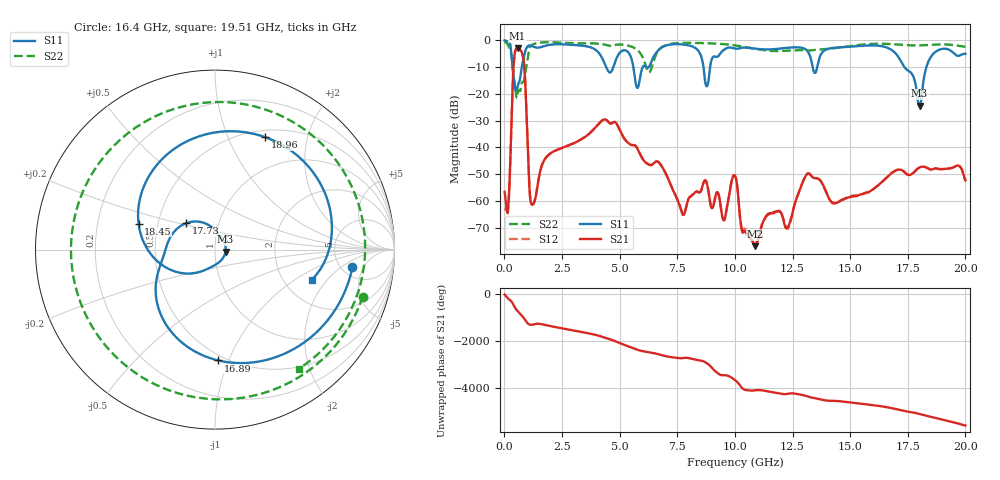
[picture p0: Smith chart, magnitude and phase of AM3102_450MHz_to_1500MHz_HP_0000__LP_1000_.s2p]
!Agilent Technologies,E8364B,MY43040894,A.07.50.67
!Agilent E8364B: A.07.50.67
!Date: Thursday, January 11, 2018 05:16:45
!Correction: S11(Full 2 Port(1,2))
!S21(Full 2 Port(1,2))
!S12(Full 2 Port(1,2))
!S22(Full 2 Port(1,2))
!S2P File: Measurements: S11, S21, S12, S22:
# Hz S  dB  R 50
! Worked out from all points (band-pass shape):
!   1601 points, 10 MHz to 20 GHz, reference 50 ohm
!   highest |S21| = -3.03 dB at 572.2 MHz (marker M1); lowest = -76.8 dB at 10.89 GHz (marker M2)
!   |S21| within 3 dB of the highest: 433.8 MHz to 803.5 MHz (369.7 MHz wide, 59.8 % of centre)
!   lowest |S11| = -24.4 dB at 18.01 GHz (marker M3), VSWR 1.13, Z = 56.2 - j1.22 ohm
!   |S11| at or under -10 dB: 355.7 MHz to 753.7 MHz (398.1 MHz wide, 71.8 % of centre); 5.595 GHz to 6.003 GHz (408.2 MHz wide, 7.04 % of centre); 17.35 GHz to 18.31 GHz (953.5 MHz wide, 5.35 % of centre)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
!   |S22| runs from -21.4 to -0.5 dB; largest |S21 - S12| = 0.0016
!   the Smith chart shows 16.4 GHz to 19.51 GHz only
!   S11 on the Smith chart (normalised r, x): 16.4 GHz: 6.26, -3.06; 16.89 GHz: 0.46, -0.92; 17.73 GHz: 0.70, +0.21; 18.45 GHz: 0.39, +0.14; 18.96 GHz: 0.58, +1.38; 19.51 GHz: 2.85, -1.40
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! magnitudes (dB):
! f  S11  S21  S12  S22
! 10 MHz  -0.1  -56.6  -62.9  -0.5
! 172.4 MHz  -0.6  -61.8  -61.5  -2.0
! 409.8 MHz  -14.2  -8.4  -8.4  -14.1
! 572.2 MHz  -17.4  -3.0  -3.0  -19.9
! 834.6 MHz  -6.7  -7.5  -7.5  -15.3
! 1.209 GHz  -2.2  -61.4  -61.3  -1.6
! 3.346 GHz  -2.0  -36.9  -36.9  -1.1
! 6.682 GHz  -3.7  -45.4  -45.4  -3.8
! 7.756 GHz  -1.6  -65.2  -64.6  -1.0
! 8.781 GHz  -17.1  -53.3  -53.2  -1.1
! 10.01 GHz  -3.1  -50.6  -50.6  -1.9
! 10.89 GHz  -3.1  -76.8  -76.2  -3.2
! 13.34 GHz  -8.6  -50.8  -50.9  -3.7
! 16.4 GHz  -2.2  -52.7  -52.7  -1.3
! 16.68 GHz  -3.0  -50.5  -50.5  -1.4
! 16.89 GHz  -4.2  -49.0  -49.0  -1.5
! 17.73 GHz  -13.2  -49.6  -49.6  -1.9
! 18.01 GHz  -24.4  -47.5  -47.4  -1.9
! 18.45 GHz  -6.9  -48.1  -48.1  -1.7
! 18.96 GHz  -3.3  -48.1  -48.1  -1.5
! 19.51 GHz  -4.9  -47.2  -47.3  -1.8
! 20 GHz  -5.0  -52.3  -52.2  -2.4
